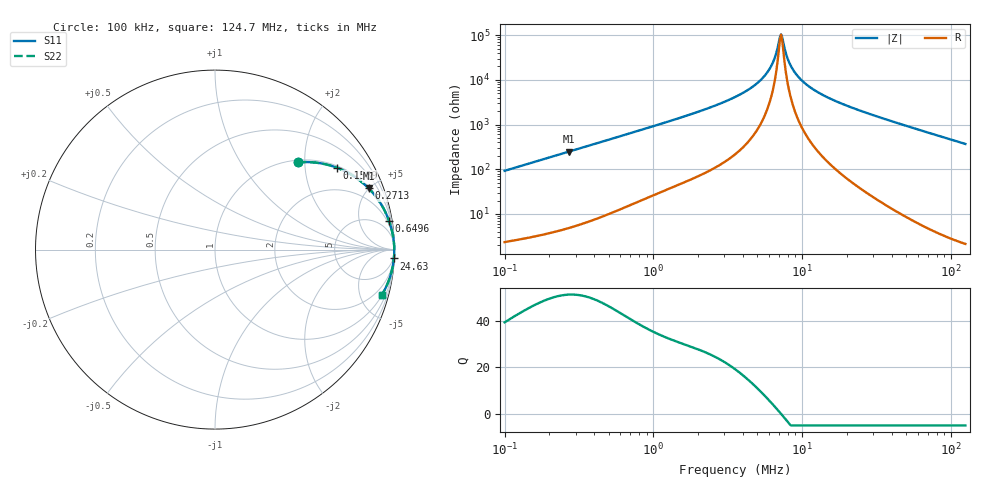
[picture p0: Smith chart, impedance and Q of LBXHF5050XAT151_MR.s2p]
! LBXHF5050XAT151_MR  S-PARAMETER MODEL  ( Standard Model )
! Model Generated by TAIYO YUDEN Corporation (http://www.ty-top.com)
! Version 1.0
! TAIYO YUDEN Control No. 20230906
! Copyright(c) 2023 TAIYO YUDEN CO.,LTD. All Rights Reserved.
! Product Description (link to TY-COMPAS)
! https://ds.yuden.co.jp/TYCOMPAS/or/detail?pn=LBXHF5050XAT151MMR&u=M
! Products Name : Inductors
! Characteristics :
!  Inductance : 150 [uH] , SRF(min) : 5.0 [MHz] , DC Resistance(max) : 1.165 [Ohm]
!  Rated Current : Saturation  470 [mA] , Temp Rise  310 [mA] (20 [degC])
!  Case Size : 5.0 x 5.0 / 0.197 x 0.197 [mm/inch] , Thickness : 3.1 / 0.122 [mm/inch]
!  (Conditions: Temperature = 25 [degC] , DC Bias Current = 0 [A])
! External Node Assignments :
!  1  o---GGG---o  2
! GND o---------o GND
! Frequency Range : 0.1MHz  -  124.6553MHz  [ 402 STEP ]
# MHz S RI R 50
! Freq[MHz].  S11 Real  S11 Imag  S21 Real  S21 Imag  S12 Real  S12 Imag  S22 Real  S22 Imag
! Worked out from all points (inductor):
!   401 points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, 100 kHz to 124.7 MHz, reference 50 ohm
!   read as one part in series: L = 146 uH near 103.6 kHz
!   highest Q = 51.2 at 271.3 kHz (marker M1), where L = 146 uH
!   self-resonance near 7.074 MHz
!   S11 on the Smith chart (normalised r, x): 100 kHz: 1.05, +1.84; 158.9 kHz: 1.06, +2.92; 271.3 kHz: 1.10, +4.97; 649.6 kHz: 1, +12; 24.63 MHz: 2, -41; 124.7 MHz: 1.04, -7.37
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0.1  0.4606 0.4859  0.5394 -0.4859  0.5394 -0.4859  0.4606 0.4859
0.158936  0.6774 0.4569  0.3226 -0.4569  0.3226 -0.4569  0.6774 0.4569
0.271269  0.856 0.3415  0.144 -0.3415  0.144 -0.3415  0.856 0.3415
0.330013  0.8967 0.2946  0.1033 -0.2946  0.1033 -0.2946  0.8967 0.2946
0.649567  0.9689 0.162  0.0311 -0.162  0.0311 -0.162  0.9689 0.162
1.089088  0.9874 0.0978  0.0126 -0.0978  0.0126 -0.0978  0.9874 0.0978
2.221438  0.9962 0.0454  0.00379 -0.0454  0.00379 -0.0454  0.9962 0.0454
3.530656  0.9982 0.0242  0.00185 -0.0242  0.00185 -0.0242  0.9982 0.0242
4.612587  0.9987 0.0144  0.00131 -0.0144  0.00131 -0.0144  0.9987 0.0144
5.611469  0.9989 0.00787  0.00109 -0.00787  0.00109 -0.00787  0.9989 0.00787
6.35699  0.999 0.0039  0.00101 -0.0039  0.00101 -0.0039  0.999 0.0039
6.949409  0.999 0.00109  0.000973 -0.00109  0.000973 -0.00109  0.999 0.00109
7.201558  0.999 -2.36e-05  0.000964 2.36e-05  0.000964 2.36e-05  0.999 -2.36e-05
7.462855  0.999 -0.00114  0.000958 0.00114  0.000958 0.00114  0.999 -0.00114
8.014236  0.999 -0.00338  0.000956 0.00338  0.000956 0.00338  0.999 -0.00338
8.761097  0.999 -0.00621  0.00097 0.00621  0.00097 0.00621  0.999 -0.00621
9.925067  0.999 -0.0103  0.00102 0.0103  0.00102 0.0103  0.999 -0.0103
11.65164  0.9989 -0.0157  0.00115 0.0157  0.00115 0.0157  0.9989 -0.0157
15.77446  0.9984 -0.0272  0.00163 0.0272  0.00163 0.0272  0.9984 -0.0272
24.62842  0.9967 -0.049  0.0033 0.049  0.0033 0.049  0.9967 -0.049
38.45196  0.9926 -0.0804  0.00744 0.0804  0.00744 0.0804  0.9926 -0.0804
124.6553  0.9301 -0.2521  0.0699 0.2521  0.0699 0.2521  0.9301 -0.2521
